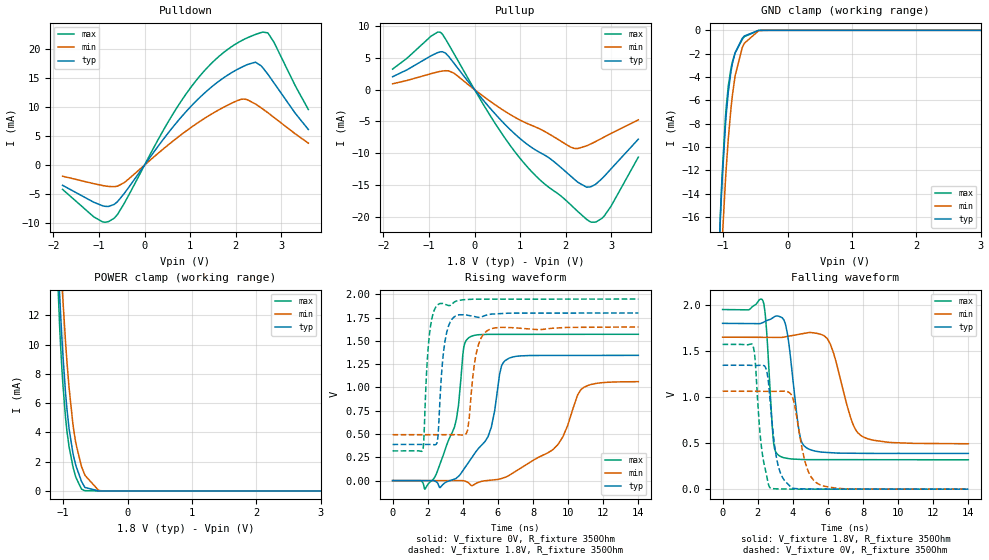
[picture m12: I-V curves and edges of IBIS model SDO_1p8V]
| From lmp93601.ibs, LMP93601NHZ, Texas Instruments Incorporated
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|   Model SDO_1p8V
[Model]   SDO_1p8V
Model_type   3-state
Polarity   Non-Inverting
Vmeas = 0.9
Vref = 1.8
Cref = 15pF
Rref = 350
|   typ   min   max
|   (nom PVT)   (fast PVT)   (slow PVT)
C_comp   0.1539p   0.1481p   0.1571p
|C_comp (ON state)   0.1677p   0.1603p   0.1688p
|C_comp (OFF state)   0.1539p   0.1481p   0.1571p
[Voltage Range]   1.8   1.65   1.95
[Temperature Range]   27   125   -25
[Pullup Reference]   1.8   1.65   1.95
[Pulldown Reference]   0   0   0
[Power Clamp Reference]   1.8   1.65   1.95
[GND Clamp Reference]   0   0   0
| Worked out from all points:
|   slope of the pulldown table from 0 to 0.27 V, typ, clamps not added: 91.4 ohm
|   slope of the pullup table from 0 to 0.27 V, typ, clamps not added: 116 ohm
|   GND clamp passes 1 mA (typ) near -0.73 V on its own axis
|   POWER clamp passes 1 mA (typ) near -0.74 V on its own axis
|   falling waveform, V_fixture 1.8V, R_fixture 350Ohm: 20-80 % time 508ps typ, 981ps min, 302ps max; typ from 1.8 V to 0.388 V
|   rising waveform, V_fixture 0V, R_fixture 350Ohm: 20-80 % time 1.45ns typ, 2.45ns min, 1ns max; typ from 0 V to 1.34 V
|   rising waveform, V_fixture 1.8V, R_fixture 350Ohm: 20-80 % time 359ps typ, 443ps min, 313ps max; typ from 0.388 V to 1.8 V
|   falling waveform, V_fixture 0V, R_fixture 350Ohm: 20-80 % time 495ps typ, 678ps min, 418ps max; typ from 1.34 V to 0 V
[Pulldown]
|   Voltage   I(typ)   I(min)   I(max)
-1.8V     -3.498mA   -1.926mA   -4.2mA
-919.8mV  -7.038mA   -3.538mA   -9.819mA
-671.4mV  -6.805mA   -3.73mA    -9.199mA
532.8mV   5.675mA    3.561mA    7.638mA
1.138V    11.09mA    7.126mA    14.64mA
1.618V    14.39mA    9.473mA    18.65mA
2.12V     16.84mA    11.34mA    21.43mA
2.434V    17.75mA    10.53mA    22.54mA
2.558V    17.12mA    9.88mA     22.86mA
2.704V    15.7mA     9.041mA    22.82mA
2.839V    14.2mA     8.228mA    21.21mA
3.595V    6.134mA    3.781mA    9.587mA
[GND Clamp]
|   Voltage   I(typ)   I(min)   I(max)
-1.8V     -173.2mA   -158.7mA   -187.9mA
-1.152V   -32.84mA   -36.5mA    -34.28mA
-1.044V   -16.26mA   -21.43mA   -15.93mA
-1.017V   -13.05mA   -18.25mA   -12.49mA
-952.2mV  -7.215mA   -11.82mA   -6.584mA
-919.8mV  -5.266mA   -9.281mA   -4.768mA
-876.6mV  -3.466mA   -6.588mA   -3.203mA
-811.8mV  -1.902mA   -3.836mA   -1.918mA
-703.8mV  -693.6uA   -1.502mA   -784.8uA
-671.4mV  -485.1uA   -1.111mA   -547uA
-396mV    -1.323uA   -12.03uA   -582nA
3.595V    0A         0A         0A
[Pullup]
|   Voltage   I(typ)   I(min)   I(max)
-1.8V     2.024mA    915.5uA    3.226mA
-957.6mV  5.312mA    2.505mA    8.393mA
-725.4mV  5.956mA    2.902mA    8.866mA
-450mV    4.129mA    2.572mA    5.632mA
354.6mV   -3.035mA   -1.895mA   -4.22mA
948.6mV   -7.389mA   -4.601mA   -10.36mA
1.424V    -9.851mA   -6.155mA   -14.12mA
2.18V     -14.03mA   -9.222mA   -18.58mA
2.455V    -15.33mA   -8.851mA   -20.38mA
2.563V    -15.24mA   -8.5mA     -20.84mA
2.844V    -13.65mA   -7.46mA    -19.89mA
3.595V    -7.795mA   -4.76mA    -10.62mA
[POWER Clamp]
|   Voltage   I(typ)   I(min)   I(max)
-1.8V     115.9mA    106.7mA    122.8mA
-1.147V   23.03mA    25.95mA    21.4mA
-1.055V   13.44mA    17.19mA    11.27mA
-1.006V   9.455mA    13.22mA    7.417mA
-963mV    6.708mA    10.18mA    5.003mA
-909mV    4.288mA    7.095mA    3.046mA
-833.4mV  2.279mA    4.102mA    1.409mA
-801mV    1.714mA    3.22mA     912.9uA
-714.6mV  646.8uA    1.665mA    122.9uA
-660.6mV  237.2uA    1.065mA    18.96uA
-412.2mV  61.16nA    15.12uA    565.3pA
3.595V    0A         0A         0A
[Ramp]
R_load = 350
|   typ   min   max
dV/dt_r   0.807139/1.45638e-09   0.637719/2.44985e-09   0.942989/1.00173e-09
dV/dt_f   0.847181/5.08365e-10   0.694225/9.80852e-10   0.978681/3.01962e-10
[Falling Waveform]
V_fixture = 1.8V
V_fixture_min = 1.65V
V_fixture_max = 1.95V
R_fixture = 350Ohm
C_fixture = 0F
|   Time   V(typ)   V(min)   V(max)
0s        1.8V       1.65V      1.95V
2.301ns   1.808V     1.648V     2.046V
2.903ns   1.866V     1.648V     512.1mV
3.301ns   1.869V     1.648V     354.8mV
3.705ns   1.676V     1.659V     333.8mV
4.384ns   601.1mV    1.682V     323.3mV
4.769ns   450.3mV    1.696V     320.7mV
6.134ns   396.4mV    1.577V     320.5mV
7.895ns   389mV      580.5mV    320.1mV
14ns      388mV      493mV      318.9mV
[Rising Waveform]
V_fixture = 0V
V_fixture_min = 0V
V_fixture_max = 0V
R_fixture = 350Ohm
C_fixture = 0F
|   Time   V(typ)   V(min)   V(max)
0s        2.349nV    13.4nV     2.768nV
2.425ns   -6.525mV   239uV      44.26mV
3.524ns   15.79mV    347.2uV    573.5mV
4.062ns   122.9mV    -2.764mV   1.44V
4.456ns   230.6mV    -48.84mV   1.548V
5.438ns   472.1mV    1.45mV     1.571V
6.406ns   1.288V     34.74mV    1.571V
9.415ns   1.344V     386mV      1.571V
10.91ns   1.345V     1.004V     1.571V
14ns      1.345V     1.063V     1.572V
[Rising Waveform]
V_fixture = 1.8V
V_fixture_min = 1.65V
V_fixture_max = 1.95V
R_fixture = 350Ohm
C_fixture = 0F
|   Time   V(typ)   V(min)   V(max)
0s        388mV      493mV      318.9mV
1.737ns   388.1mV    493mV      336.7mV
2.09ns    388.1mV    493mV      1.554V
2.62ns    567.9mV    493.1mV    1.895V
2.984ns   1.495V     493.1mV    1.894V
3.589ns   1.768V     492.7mV    1.925V
4.276ns   1.776V     542.4mV    1.945V
4.751ns   1.759V     1.351V     1.949V
5.35ns    1.778V     1.605V     1.949V
14ns      1.8V       1.65V      1.95V
[Falling Waveform]
|Gnd
V_fixture = 0V
V_fixture_min = 0V
V_fixture_max = 0V
R_fixture = 350Ohm
C_fixture = 0F
|   Time   V(typ)   V(min)   V(max)
0s        1.345V     1.063V     1.572V
1.737ns   1.343V     1.062V     1.553V
2.233ns   1.346V     1.062V     427.7mV
2.53ns    1.27V      1.062V     129.4mV
2.716ns   947.1mV    1.062V     13.13mV
3.182ns   242.4mV    1.062V     2.837mV
3.989ns   12.21mV    995.1mV    644.3uV
4.751ns   2.459mV    264.7mV    595.3uV
5.542ns   942.3uV    48.01mV    544.3uV
14ns      1.216uV    6.257uV    -77.48nV
